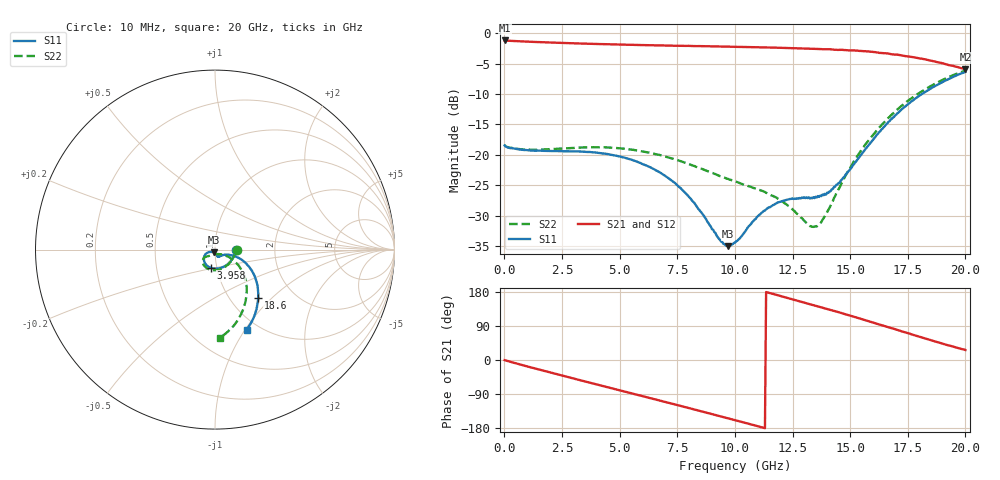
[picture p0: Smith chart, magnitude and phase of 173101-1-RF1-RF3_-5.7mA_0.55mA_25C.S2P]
!  2-Port S-parameters saved by WinCal
! VAR MeasName=S-Parameters (CALIBRATED_DATA) read from VNA (N5242A)
! VAR MeasDate=2017-7-20 9:25:04
! VAR NAME=173101-1-RF1-RF3_-5.7mA_0.55mA_25C
! VAR FILENAME=173101-1-RF1-RF3_-5.7mA_0.55mA_25C.S2P
! VAR DATE=2017-7-20 9:25:04
! VAR PHYS_PORTS=1,2
# Hz S DB R 50
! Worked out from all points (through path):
!   401 points, 10 MHz to 20 GHz, reference 50 ohm
!   highest |S21| = -1.19 dB at 10 MHz (marker M1); lowest = -5.9 dB at 20 GHz (marker M2)
!   group delay of S21, straight-line fit = 45.9 ps
!   lowest |S11| = -35.0 dB at 9.705 GHz (marker M3), VSWR 1.04, Z = 49.2 - j1.58 ohm
!   |S11| at or under -10 dB: start of sweep to 18.11 GHz
!   |S22| runs from -31.8 to -6.2 dB; largest |S21 - S12| = 0.0076
!   S11 on the Smith chart (normalised r, x): 10 MHz: 1.27, -0.00; 3.958 GHz: 0.94, -0.19; 18.6 GHz: 1.34, -0.83; 20 GHz: 0.87, -1.02
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1e7  -18.46 -0.8  -1.19 -0.3  -1.19 -0.3  -18.38 -0.8
1.559225e9  -19.31 -48.4  -1.47 -26.1  -1.47 -26.1  -19.13 -47.4
3.358325e9  -19.47 -90.8  -1.71 -54.5  -1.70 -54.4  -18.79 -86.9
3.958025e9  -19.62 -102.9  -1.77 -63.8  -1.77 -63.8  -18.75 -97.6
5.457275e9  -20.73 -129.2  -1.91 -87.0  -1.91 -87.0  -19.12 -119.5
6.70665e9  -22.80 -146.8  -2.00 -106.6  -1.99 -106.4  -19.99 -133.0
7.956025e9  -26.69 -157.8  -2.08 -126.1  -2.10 -126.0  -21.46 -141.4
9.30535e9  -33.80 -137.8  -2.18 -147.5  -2.18 -147.5  -23.43 -142.8
9.70515e9  -35.02 -115.5  -2.21 -153.9  -2.20 -153.9  -23.96 -141.9
1.0005e10  -34.43 -98.3  -2.24 -158.7  -2.24 -158.7  -24.34 -140.6
1.105448e10  -29.87 -72.3  -2.31 -175.8  -2.32 -175.6  -25.77 -135.7
1.175412e10  -28.06 -69.7  -2.37 172.7  -2.38 172.9  -26.94 -131.1
1.24038e10  -27.25 -68.7  -2.44 161.9  -2.43 162.0  -28.61 -123.4
1.335332e10  -27.15 -57.9  -2.56 145.9  -2.54 145.9  -31.83 -88.5
1.38031e10  -26.53 -47.2  -2.64 138.0  -2.64 138.1  -30.66 -58.0
1.445278e10  -24.85 -31.8  -2.74 126.9  -2.75 127.1  -25.93 -34.6
1.525238e10  -21.09 -20.0  -2.86 112.6  -2.85 112.8  -20.54 -28.5
1.590205e10  -17.96 -18.8  -3.04 100.5  -3.05 100.5  -17.13 -32.0
1.670165e10  -14.48 -24.0  -3.38 85.7  -3.42 85.7  -13.79 -39.9
1.76012e10  -11.40 -34.4  -3.85 69.2  -3.84 69.4  -10.86 -51.8
1.86007e10  -8.86 -48.1  -4.61 50.5  -4.64 50.8  -8.47 -66.2
2e10  -6.37 -68.6  -5.91 26.3  -5.94 26.9  -6.15 -86.9
